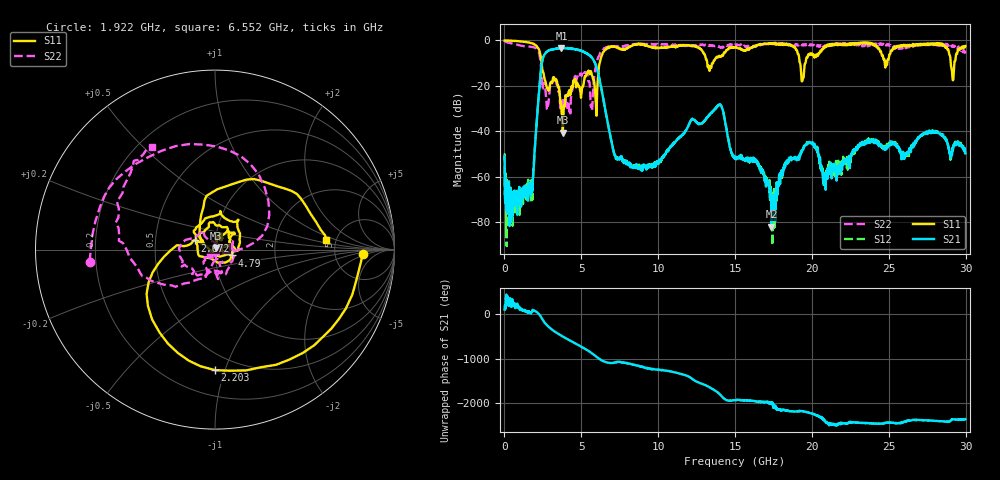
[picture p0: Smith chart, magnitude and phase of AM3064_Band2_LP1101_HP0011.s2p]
# Hz S DB R 50.0
!freq dBS11 angS11 dBS21 angS21 dBS12 angS12 dBS22 angS22
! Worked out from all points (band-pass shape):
!   1600 points, 10 MHz to 29.98 GHz, reference 50 ohm
!   highest |S21| = -3.31 dB at 3.703 GHz (marker M1); lowest = -82.0 dB at 17.37 GHz (marker M2)
!   |S21| within 3 dB of the highest: 2.598 GHz to 5.464 GHz (2.866 GHz wide, 71.1 % of centre)
!   lowest |S11| = -40.5 dB at 3.796 GHz (marker M3), VSWR 1.02, Z = 50.6 + j0.704 ohm
!   |S11| at or under -10 dB: 2.414 GHz to 6.196 GHz (3.781 GHz wide, 87.8 % of centre); 13.19 GHz to 13.57 GHz (378.7 MHz wide, 2.83 % of centre); 19.23 GHz to 19.58 GHz (347.9 MHz wide, 1.79 % of centre)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
!   |S22| runs from -32.2 to -0.2 dB; largest |S21 - S12| = 0.021
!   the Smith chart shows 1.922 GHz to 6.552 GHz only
!   S11 on the Smith chart (normalised r, x): 1.922 GHz: 10, -1; 2.203 GHz: 0.38, -0.93; 2.672 GHz: 0.80, +0.08; 4.79 GHz: 1.20, -0.08; 6.552 GHz: 4.17, +0.69
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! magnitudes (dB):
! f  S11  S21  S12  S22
! 10 MHz  0.0  -51.0  -49.8  -0.2
! 591.1 MHz  -0.2  -66.8  -73.3  -1.5
! 1.922 GHz  -1.7  -54.0  -53.1  -3.1
! 2.203 GHz  -3.5  -26.5  -26.5  -4.8
! 2.672 GHz  -18.2  -5.5  -5.5  -22.1
! 3.703 GHz  -29.2  -3.3  -3.4  -26.5
! 3.796 GHz  -40.5  -3.4  -3.3  -29.0
! 4.79 GHz  -20.1  -4.3  -4.1  -16.1
! 5.015 GHz  -23.0  -4.7  -4.7  -15.7
! 5.671 GHz  -15.0  -7.5  -7.5  -29.7
! 5.952 GHz  -28.5  -11.1  -11.1  -10.9
! 6.552 GHz  -4.1  -30.4  -30.4  -3.5
! 7.283 GHz  -3.1  -51.6  -51.3  -2.6
! 10 GHz  -3.4  -53.2  -52.8  -1.8
! 13.97 GHz  -7.0  -28.5  -28.3  -2.9
! 15 GHz  -2.9  -52.2  -51.5  -1.9
! 17.37 GHz  -1.5  -82.0  -68.5  -1.2
! 19.37 GHz  -17.9  -48.3  -48.3  -2.1
! 19.99 GHz  -5.7  -45.5  -45.1  -1.7
! 20.87 GHz  -2.6  -64.1  -58.5  -2.8
! 25 GHz  -8.0  -46.1  -46.0  -1.8
! 29.98 GHz  -2.5  -49.7  -48.6  -4.5
